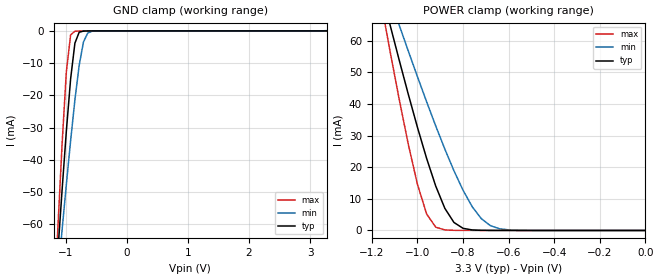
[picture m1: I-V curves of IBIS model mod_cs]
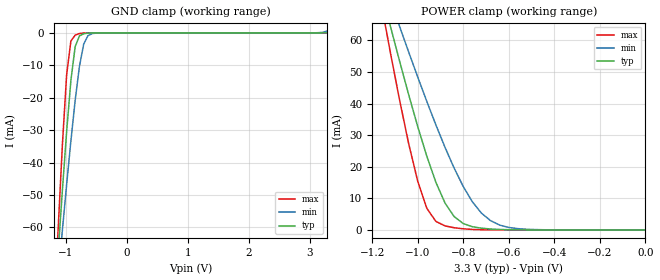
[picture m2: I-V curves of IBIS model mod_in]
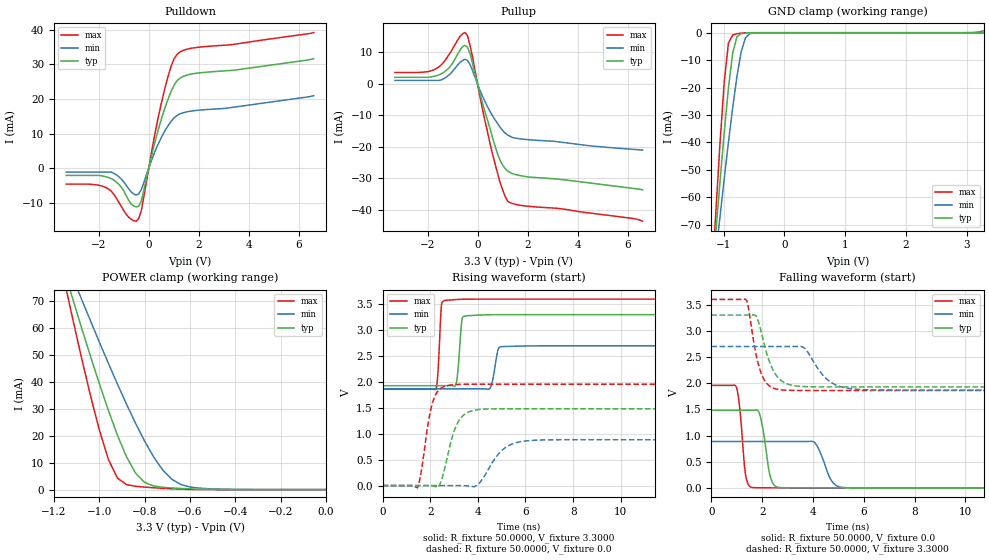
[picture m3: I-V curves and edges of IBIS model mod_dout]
| IBIS (I/O, Buffer, Information, Specification) Model, officially
| electronic behavioral standard for Buffer structures of digital pins.
[IBIS ver]  4.0
[File name] rhfad128_3v3_rev1.ibs
[File Rev]  1.0
[Date]   20 Nov 2018
[Source]   CAD & Design Services (Catania) - STMicroelectronics
[Notes]
   (Note1)  This IBIS model is the model of the product with package
   (Flat16 package elements);
   (Note2)  This IBIS model is extracted with nominal 3.3V power supply
   (min:2.7V, typ:3.3V, max:3.6V);
   (Note3)  This IBIS model has some Notes about the non-monotonicity
   of the I-V curves, but they are not indicative of problems
   inside the model;
[Disclaimer]
   Customers are solely responsible for all aspects of their
   own product designs or applications using this IBIS Model.
   STMicroelectronics assumes no liability for Custmer Designs
   and applications associated to this IBIS Model.
   In the use of this IBIS Model Customer shall not modify,
   disassemble, alter this Model in whole or in part.
   If Customers do not accept these terms, the IBIS Model
   may not be used. For any problems or modifications please
   contact STMicroelectronics (www.st.com).
[Copyright] (c) 2018 STMicroelectronics
|   Component RHFAD128
[Component] RHFAD128
[Manufacturer] STMicroelectronics
[Package]
| variable  typ   min   max
R_pkg   0.0   0.0   0.0
L_pkg   0.0H   0.0H   0.0H
C_pkg   0.0F   0.0F   0.0F
[Pin]  signal_name   model_name   R_pin   L_pin   C_pin
1   CS   mod_cs   0.0   0.0   0.0
2   AVCC   POWER   0.0   0.0   0.0
3   AGND   GND   0.0   0.0   0.0
4   IN0   mod_in   0.0   0.0   0.0
5   IN1   mod_in   0.0   0.0   0.0
6   IN2   mod_in   0.0   0.0   0.0
7   IN3   mod_in   0.0   0.0   0.0
8   IN4   mod_in   0.0   0.0   0.0
9   IN5   mod_in   0.0   0.0   0.0
10   IN6   mod_in   0.0   0.0   0.0
11   IN7   mod_in   0.0   0.0   0.0
12   DGND   GND   0.0   0.0   0.0
13   DVCC   POWER   0.0   0.0   0.0
14   DIN   mod_din   0.0   0.0   0.0
15   DOUT   mod_dout   0.0   0.0   0.0
16   SCK   mod_ck   0.0   0.0   0.0
[Package Model]  292130_PKG_IBIS
[Define Package Model]  292130_PKG_IBIS
[Manufacturer]  STMicroelectronics
[OEM]  STMicroelectronics
[Description]  ceramic flat-16
[Number Of Pins] 16
[Pin Numbers]
|Pin Num   Terminal Name
1   | NET1:bwpad1_source
2   | NET2:bwpad2_source
3   | NET3:bwpad6_source
4   | NET4:bwpad7_source
5   | NET5:bwpad8_source
6   | NET6:bwpad12_source
7   | NET7:bwpad13_source
8   | NET8:net8_source
9   | NET9:bwpad19_source
10   | NET10:bwpad20_source
11   | NET11:bwpad24_source
12   | NET12:bwpad25_source
13   | NET13:bwpad26_source
14   | NET14:bwpad30_source
15   | NET15:bwpad31_source
16   | NET16:net16_source
[Model Data]
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[End Model Data]
[End Package Model]
| Models and submodels in the file (5): mod_cs (Input), mod_in (Input), mod_dout (3-state), mod_din (Input), mod_ck (Input)
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|   Model mod_cs
[Model]   mod_cs
Model_type Input
Vinl   =   0.800V
Vinh   =   2.100V
|C_comp   0.223pF   0.213pF   0.243pF
C_comp   3.500pF   3.450pF   3.550pF
[Temperature Range]  25.0000   0.1250k   -55.0000
[Voltage Range]   3.3000V   2.7000V   3.6000V
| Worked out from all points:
|   GND clamp passes 1 mA (typ) near -0.79 V on its own axis
|   POWER clamp passes 1 mA (typ) near -0.81 V on its own axis
[GND_clamp]
|Voltage   I(typ)   I(min)   I(max)
-3.3V     -733.3mA   -563.6mA   -997.2mA
-1.2V     -88.89mA   -91.27mA   -89.53mA
-1.13V    -68.87mA   -76.43mA   -61.64mA
-1.06V    -49.45mA   -61.85mA   -35.25mA
-990mV    -31.08mA   -47.66mA   -12.67mA
-920mV    -14.89mA   -34.06mA   -1.24mA
-850mV    -3.806mA   -21.45mA   -93.51uA
-780mV    -413.8uA   -10.7mA    -38.58uA
-710mV    -52.85uA   -3.454mA   -18.15uA
-640mV    -15.91uA   -659.6uA   -5.906uA
-570mV    -5.522uA   -101.6uA   -1.093uA
3.28V     6.546pA    105.3uA    5.6pA
[POWER_clamp]
|Voltage   I(typ)   I(min)   I(max)
-3.28V    725.8mA    557.9mA    987.1mA
-1.16V    76.26mA    81.66mA    72.25mA
-1.12V    64.93mA    73.23mA    56.56mA
-1.08V    53.82mA    64.9mA     41.42mA
-1V       32.59mA    48.61mA    14.57mA
-960mV    22.82mA    40.72mA    5.252mA
-920mV    14.06mA    33.07mA    1.048mA
-880mV    7.005mA    25.74mA    169.8uA
-840mV    2.538mA    18.89mA    49.5uA
-720mV    51.97uA    3.735mA    13.74uA
-640mV    13.8uA     536.4uA    4.816uA
0V        6.718pA    87.64pA    7.2pA
|   Model mod_in
[Model]   mod_in   | *the IN0-IN7 are analog inputs
Model_type Input
Vinl   =   0.100V
Vinh   =   3.200V
C_comp   1.306pF   1.292pF   1.358pF
[Temperature Range]  25.0000   0.1250k   -55.0000
[Voltage Range]   3.3000V   2.7000V   3.6000V
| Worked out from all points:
|   GND clamp passes 1 mA (typ) near -0.78 V on its own axis
|   POWER clamp passes 1 mA (typ) near -0.76 V on its own axis
[GND_clamp]
|Voltage   I(typ)   I(min)   I(max)
-3.3V     -732mA     -562.4mA   -995.8mA
-1.13V    -67.94mA   -75.42mA   -60.79mA
-1.06V    -48.63mA   -60.89mA   -34.71mA
-990mV    -30.46mA   -46.76mA   -12.9mA
-920mV    -14.65mA   -33.25mA   -2.48mA
-850mV    -4.225mA   -20.8mA    -700.8uA
-780mV    -923.7uA   -10.32mA   -190.1uA
-710mV    -261.8uA   -3.459mA   -37.71uA
-640mV    -72.84uA   -834.8uA   -5.445uA
-570mV    -17.3uA    -211.4uA   -567.6nA
3.07V     574.3pA    16.91uA    498.2pA
3.28V     636.3pA    573.4uA    544.2pA
[POWER_clamp]
|Voltage   I(typ)   I(min)   I(max)
-3.28V    724.4mA    556.6mA    985.6mA
-1.16V    75.67mA    81.05mA    71.61mA
-1.12V    64.47mA    72.7mA     56.11mA
-1.08V    53.5mA     64.45mA    41.24mA
-1V       32.73mA    48.39mA    15.43mA
-960mV    23.32mA    40.65mA    6.846mA
-920mV    15.04mA    33.19mA    2.692mA
-880mV    8.509mA    26.11mA    1.29mA
-800mV    2.019mA    13.75mA    366uA
-720mV    564.4uA    5.321mA    73.81uA
-600mV    75.39uA    794.8uA    3.298uA
0V        645.8pA    16.33nA    614.6pA
|   Model mod_dout
[Model]   mod_dout
Model_type 3-state
Enable   Active-Low
Polarity   Inverting
|Vinl   =   0.800V
|Vinh   =   2.100V
Vmeas  =   1.650V
Cref   =   50pf
|C_comp   0.404pF   0.385pF   0.443pF
C_comp   1.950pF   1.940pF   1.960pF
[Temperature Range]  25.0000   0.1250k   -55.0000
[Voltage Range]   3.3000V   2.7000V   3.6000V
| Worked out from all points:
|   slope of the pulldown table from 0 to 0.495 V, typ, clamps not added: 35.6 ohm
|   slope of the pullup table from 0 to 0.495 V, typ, clamps not added: 35.1 ohm
|   GND clamp passes 1 mA (typ) near -0.75 V on its own axis
|   POWER clamp passes 1 mA (typ) near -0.73 V on its own axis
|   rising waveform, R_fixture 50.0000, V_fixture 3.3000: 20-80 % time 132ps typ, 183ps min, 110ps max; typ from 1.93 V to 3.3 V
|   rising waveform, R_fixture 50.0000, V_fixture 0.0: 20-80 % time 534ps typ, 813ps min, 411ps max; typ from 0 V to 1.48 V
|   falling waveform, R_fixture 50.0000, V_fixture 0.0: 20-80 % time 275ps typ, 426ps min, 201ps max; typ from 1.48 V to 0 V
|   falling waveform, R_fixture 50.0000, V_fixture 3.3000: 20-80 % time 546ps typ, 785ps min, 425ps max; typ from 3.3 V to 1.93 V
[Pulldown]
|Voltage   I(typ)   I(min)   I(max)
-3.3V     -2.1mA     -1.122mA   -4.588mA
-1.7V     -2.51mA    -1.122mA   -5.633mA
-1.2V     -4.61mA    -2.442mA   -9.823mA
-800mV    -9.289mA   -5.972mA   -14.19mA
-500mV    -11.19mA   -7.769mA   -15.35mA
-300mV    -9.527mA   -6.234mA   -12.4mA
200mV     6.145mA    3.924mA    8.124mA
600mV     16.33mA    10.18mA    21.7mA
900mV     22.24mA    13.58mA    29.52mA
1.1V      24.93mA    15.06mA    32.55mA
1.8V      27.3mA     16.58mA    34.74mA
6.6V      31.62mA    20.95mA    39.16mA
[Pullup]
|Voltage   I(typ)   I(min)   I(max)
-3.3V     2.1mA      1.122mA    3.626mA
-1.6V     2.713mA    1.122mA    5.11mA
-1.1V     5.432mA    3.131mA    9.844mA
-700mV    10.75mA    6.852mA    15.15mA
-500mV    12.27mA    7.869mA    16.34mA
-400mV    11.65mA    7.426mA    15.38mA
-300mV    9.667mA    6.234mA    12.3mA
300mV     -8.946mA   -5.68mA    -11.84mA
800mV     -22.25mA   -12.58mA   -28.4mA
1.2V      -27.71mA   -16.25mA   -37.29mA
2V        -29.58mA   -17.74mA   -38.93mA
6.6V      -33.7mA    -21.07mA   -43.73mA
[GND_clamp]
|Voltage   I(typ)   I(min)   I(max)
-3.3V     -734.6mA   -565.5mA   -998.1mA
-1.2V     -93.3mA    -96.28mA   -93.71mA
-1.13V    -73.66mA   -81.71mA   -66.46mA
-1.06V    -54.63mA   -67.39mA   -40.76mA
-990mV    -36.56mA   -53.44mA   -18.21mA
-920mV    -20.19mA   -40mA      -3.721mA
-850mV    -7.396mA   -27.32mA   -816.7uA
-780mV    -1.457mA   -15.93mA   -365.6uA
-710mV    -358.4uA   -6.908mA   -126.5uA
-640mV    -121.8uA   -1.871mA   -26.87uA
-570mV    -33.88uA   -376.9uA   -3.684uA
3.28V     24.44pA    718.4uA    20.16pA
[POWER_clamp]
|Voltage   I(typ)   I(min)   I(max)
-3.28V    728.3mA    561mA      988.9mA
-1.16V    82.72mA    87.62mA    79.81mA
-1.12V    71.53mA    79.26mA    64.45mA
-1.08V    60.53mA    70.99mA    49.56mA
-1V       39.36mA    54.76mA    22.27mA
-960mV    29.42mA    46.85mA    11.29mA
-920mV    20.21mA    39.14mA    4.304mA
-840mV    6.112mA    24.59mA    1.233mA
-800mV    2.682mA    17.97mA    923.3uA
-680mV    608.6uA    3.818mA    296.4uA
-600mV    280.9uA    960.7uA    79.24uA
0V        28.33pA    1.052nA    28.8pA
[Ramp]
| variable   typ   min   max
dV/dt_r   2.0/1.4n   1.0/1.30n   2.20/2.0n
dV/dt_f   2.0/1.4n   1.0/1.30n   2.20/2.0n
R_load = 50.0000
[Rising Waveform]
R_fixture= 50.0000
V_fixture= 3.3000
V_fixture_min= 2.7000
V_fixture_max= 3.6000
|time   V(typ)   V(min)   V(max)
0s        1.928V     1.868V     1.86V
2.24ns    1.928V     1.868V     1.859V
2.46ns    1.928V     1.868V     3.43V
2.62ns    1.928V     1.868V     3.575V
3.08ns    1.951V     1.868V     3.592V
3.32ns    3.165V     1.868V     3.597V
3.44ns    3.272V     1.868V     3.598V
4.5ns     3.298V     1.87V      3.6V
4.98ns    3.3V       2.681V     3.6V
15ns      3.3V       2.699V     3.6V
[Rising Waveform]
R_fixture= 50.0000
V_fixture= 0.0
V_fixture_min= 0.0
V_fixture_max= 0.0
|time   V(typ)   V(min)   V(max)
0s        8.739nV    82.97nV    -10.14nV
1.46ns    -120.1nV   105.2nV    -44.1mV
2.1ns     -7.221mV   105.5nV    1.608V
2.4ns     15.6mV     109.6nV    1.861V
2.68ns    470.3mV    66.88nV    1.926V
3.16ns    1.217V     -9.142uV   1.953V
3.86ns    1.456V     -22.87mV   1.957V
4.92ns    1.482V     638.9mV    1.957V
5.88ns    1.483V     854.2mV    1.957V
15ns      1.483V     885.2mV    1.957V
[Falling Waveform]
R_fixture= 50.0000
V_fixture= 0.0
V_fixture_min= 0.0
V_fixture_max= 0.0
|time   V(typ)   V(min)   V(max)
0s        1.483V     885.2mV    1.957V
980ps     1.483V     885.2mV    1.928V
1.34ns    1.483V     885.2mV    258.6mV
1.58ns    1.483V     885.2mV    9.454mV
1.9ns     1.406V     885.2mV    1.658mV
2.3ns     244.7mV    885.2mV    258.4uV
2.62ns    9.795mV    885.2mV    60.39uV
4.02ns    48.79uV    880.9mV    -226.6nV
5.14ns    1.157uV    8.278mV    -345.5nV
15ns      -1.346nV   109nV      127.9nV
[Falling Waveform]
R_fixture= 50.0000
V_fixture= 3.3000
V_fixture_min= 2.7000
V_fixture_max= 3.6000
|time   V(typ)   V(min)   V(max)
0s        3.3V       2.7V       3.6V
1.4ns     3.3V       2.7V       3.568V
1.76ns    3.286V     2.7V       2.543V
1.92ns    3.057V     2.7V       2.242V
2.24ns    2.472V     2.7V       1.964V
2.56ns    2.145V     2.7V       1.887V
3.6ns     1.936V     2.69V      1.86V
4.52ns    1.929V     2.087V     1.86V
5.48ns    1.928V     1.895V     1.86V
15ns      1.928V     1.868V     1.86V
